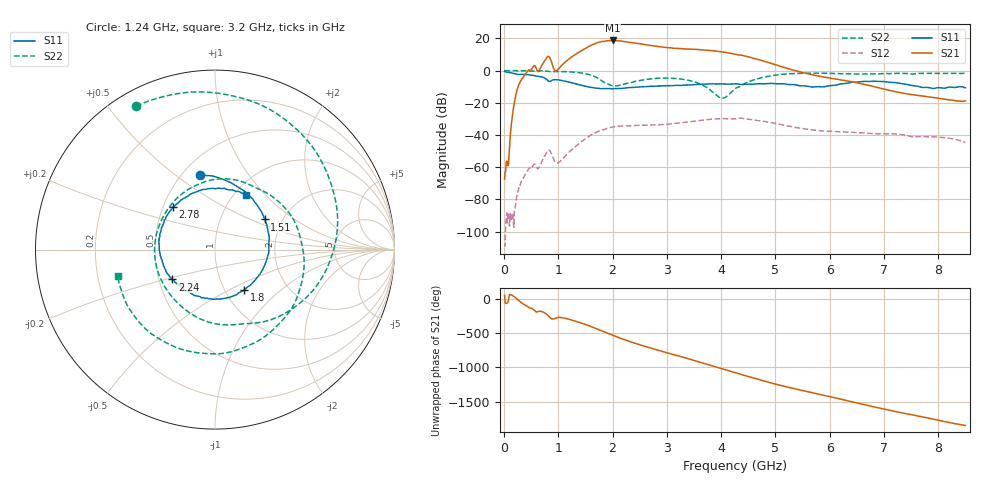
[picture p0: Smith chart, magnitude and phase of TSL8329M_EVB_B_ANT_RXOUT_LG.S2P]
!Agilent Technologies,E5071C,MY46523237,B.13.01
!Date: Tue Aug 02 11:41:58 2022
!Data & Calibration Information:
!Freq	S11:SOLT2(ON)	S21:SOLT2(ON)	S12:SOLT2(ON)	S22:SOLT2(ON)
!PortZ  Port1:50+j0  Port2:50+j0
!Above PortZ is port z conversion or system Z0 setting when saving the data.
!When reading, reference impedance value at option line is always used.
# Hz S dB R 50
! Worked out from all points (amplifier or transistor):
!   850 points, 10 MHz to 8.5 GHz, reference 50 ohm
!   highest |S21| = 18.8 dB at 2 GHz (marker M1)
!   |S21| within 3 dB of that: 1.602 GHz to 2.676 GHz (1.074 GHz wide, 50.2 % of centre)
!   unconditionally stable (mu >= 1): 13.96 MHz to end of sweep
!   at 1.42 GHz: K = 5.12, MAG = 18.2 dB, |S12| = -44.3 dB
!   at 4.26 GHz: K = 3.77, MAG = 11.4 dB, |S12| = -30.0 dB
!   at 8.5 GHz: K = 214.77, MAG = -13.5 dB, |S12| = -44.5 dB
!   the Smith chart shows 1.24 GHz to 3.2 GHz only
!   S11 on the Smith chart (normalised r, x): 1.24 GHz: 0.61, +0.62; 1.51 GHz: 1.62, +0.61; 1.8 GHz: 1.23, -0.60; 2.24 GHz: 0.59, -0.21; 2.78 GHz: 0.56, +0.30; 3.2 GHz: 1.12, +0.78
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1e7  -0.30 -4.8  -67.32 53.2  -107.71 26.2  0.01 -2.0
2.6e8  -2.34 -62.3  -9.83 -15.3  -74.74 -171.8  -0.03 -52.0
7.6e8  -4.82 -171.2  6.78 153.1  -52.33 45.1  -0.22 -148.0
1.24e9  -7.42 101.0  8.39 55.6  -49.27 -27.0  -0.80 118.8
1.43e9  -9.05 53.8  12.48 8.0  -44.00 -61.8  -1.45 73.0
1.51e9  -9.78 31.3  14.13 -14.1  -42.07 -79.6  -1.95 50.8
1.65e9  -10.62 -10.0  16.45 -56.5  -39.11 -114.9  -3.37 5.3
1.8e9  -11.17 -54.0  18.10 -105.7  -36.95 -157.6  -6.27 -55.6
2e9  -11.24 -103.1  18.77 -169.3  -35.03 147.1  -9.33 -157.1
2.24e9  -10.74 -145.1  17.97 119.4  -34.23 82.5  -8.05 85.2
2.53e9  -9.96 171.5  16.55 44.1  -33.91 13.6  -5.93 -10.9
2.78e9  -9.56 134.6  15.28 -15.2  -33.74 -41.6  -4.86 -76.6
2.84e9  -9.49 125.2  15.01 -28.7  -33.64 -54.3  -4.72 -90.4
3.2e9  -9.12 60.9  13.81 -108.5  -32.62 -128.7  -5.00 -164.6
3.51e9  -8.66 -1.8  13.24 -178.4  -31.36 165.8  -6.96 141.3
3.81e9  -8.17 -56.8  12.53 110.6  -30.17 98.7  -12.28 99.9
4.26e9  -8.19 -115.0  10.20 2.8  -30.00 -3.4  -11.20 112.9
4.55e9  -8.40 -142.1  8.15 -65.2  -30.39 -71.1  -6.32 53.7
4.9e9  -7.95 -176.8  4.77 -142.8  -32.14 -145.1  -3.35 -26.1
5.67e9  -10.16 64.3  -2.49 71.2  -36.75 67.9  -1.53 -154.7
7.09e9  -7.06 -175.2  -12.14 174.1  -39.18 162.7  -1.91 -47.6
8.5e9  -10.64 -88.9  -18.78 -49.2  -44.51 -68.5  -1.68 104.9
